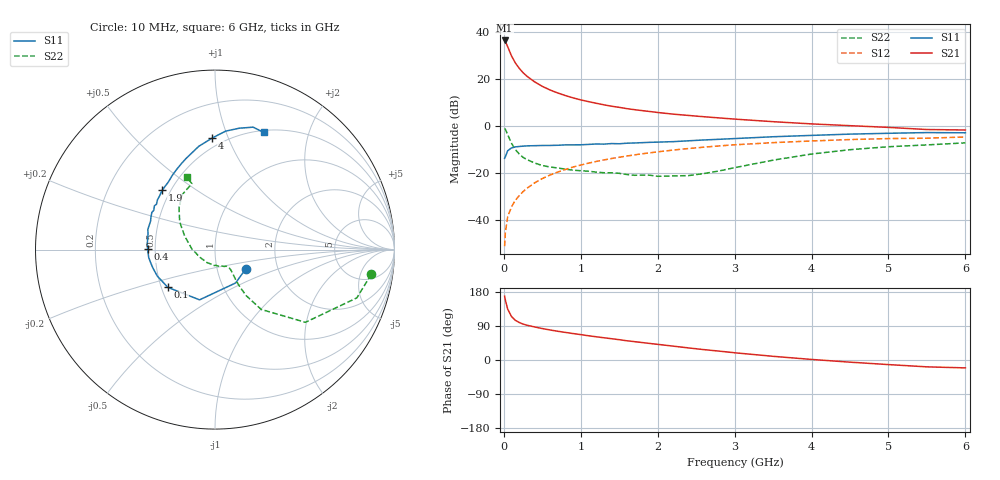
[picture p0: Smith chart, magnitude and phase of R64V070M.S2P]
! SIEMENS Small Signal Semiconductors
! BFR193
! Si NPN RF Bipolar Junction Transistor in SOT23
! VCE = 4 V  IC = 70 mA
! Common Emitter S-Parameters:  May  1996
# GHz  S  MA  R  50
!  f  S11  S21  S12  S22
! GHz  MAG  ANG  MAG  ANG  MAG  ANG  MAG  ANG
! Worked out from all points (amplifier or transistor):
!   36 points, 10 MHz to 6 GHz, reference 50 ohm
!   highest |S21| = 36.4 dB at 10 MHz (marker M1)
!   |S21| within 3 dB of that: start of sweep to 54.22 MHz
!   unconditionally stable (mu >= 1): 327.3 MHz to 2.1 GHz
!   at 250 MHz: K = 0.98, MSG = 25.4 dB, |S12| = -28.1 dB
!   at 1.4 GHz: K = 1.02, MAG = 10.3 dB, |S12| = -14.0 dB
!   at 6 GHz: K = 0.96, MSG = 1.5 dB, |S12| = -4.8 dB
!   S11 on the Smith chart (normalised r, x): 10 MHz: 1.37, -0.31; 100 MHz: 0.54, -0.26; 400 MHz: 0.45, +0.00; 1.9 GHz: 0.45, +0.37; 4 GHz: 0.43, +0.88; 6 GHz: 0.52, +1.36
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0.01  0.2023 -32.4  65.85 168.4  0.0027 83.5  0.8811 -9.0
0.02  0.2185 -58.3  62.59 157.8  0.0053 76.1  0.8348 -18.8
0.05  0.2929 -107.1  48.45 134.2  0.0114 70.4  0.6465 -38.8
0.1  0.3368 -141.4  30.71 114.6  0.0187 71.0  0.4214 -52.3
0.15  0.3538 -155.5  21.78 104.6  0.0258 71.9  0.3093 -55.9
0.2  0.3608 -163.4  16.78 99.0  0.0322 73.6  0.2497 -56.3
0.25  0.3669 -169.3  13.53 94.8  0.0394 74.5  0.2113 -55.8
0.3  0.372 -173.3  11.38 91.8  0.0463 75.5  0.19 -54.9
0.4  0.3753 179.7  8.63 87.2  0.0604 75.6  0.1604 -53.1
0.5  0.3789 175.2  6.916 83.0  0.0746 75.5  0.1415 -52.1
0.6  0.3798 170.8  5.794 79.3  0.0889 74.4  0.1319 -52.1
0.7  0.3831 166.8  4.999 75.8  0.1028 73.5  0.1255 -53.0
0.9  0.3909 159.9  3.928 69.8  0.1313 70.9  0.1126 -55.4
1.1  0.3994 153.4  3.266 64.0  0.1589 68.2  0.1072 -61.3
1.4  0.4165 144.2  2.609 56.2  0.1998 63.8  0.0991 -71.4
1.9  0.4426 131.5  2.008 43.6  0.2653 56.2  0.088 -100.3
2.2  0.4576 124.6  1.767 36.6  0.3025 51.5  0.0849 -121.0
3.5  0.5821 99.0  1.22 9.7  0.4358 30.7  0.1843 156.1
4  0.6221 91.4  1.094 1.5  0.4732 23.7  0.2491 142.1
4.5  0.6625 84.9  1.003 -5.7  0.507 16.6  0.3085 130.6
5.5  0.7145 72.7  0.83 -18.1  0.5421 2.9  0.3897 109.3
6  0.7069 67.4  0.811 -20.8  0.5754 -1.1  0.4312 111.3
